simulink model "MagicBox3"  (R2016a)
settings: Solver=VariableStepAuto  StartTime=0.0  StopTime=inf  RelTol=1e-3

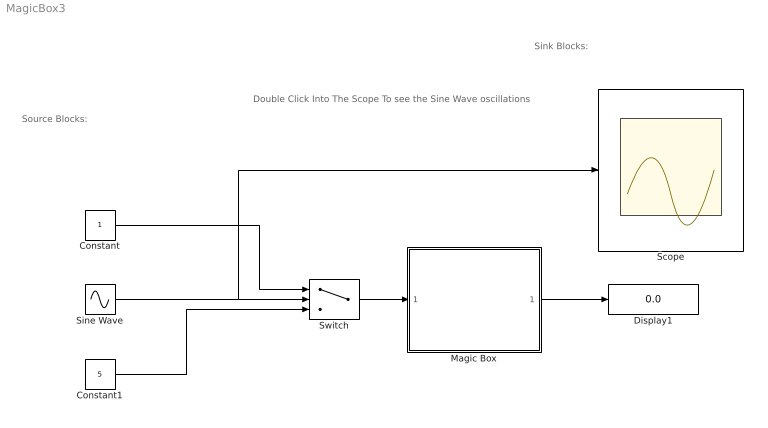
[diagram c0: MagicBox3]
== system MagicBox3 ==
  note: Double Click Into The Scope To see the Sine Wave oscillations
  note: Sink Blocks:
  note: Source Blocks:
  Constant : Constant
  Constant1 : Constant  Value=5
  Display1 : Display
  Magic Box : MATLAB Function  TreatAsAtomicUnit=on
  Scope : Scope
  Sine Wave : Sin  SampleTime=0
  Switch : Switch  Criteria=u2 > Threshold
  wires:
  Constant/1 -> Switch/1
  Magic Box/1(output) -> Display1/1
  Constant1/1 -> Switch/3
  Switch/1 -> Magic Box/1(input)
  Sine Wave/1 -> Scope/1, Switch/2

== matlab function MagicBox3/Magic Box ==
function output = MagicBox(input)
number = input;
output = number+1;
end
